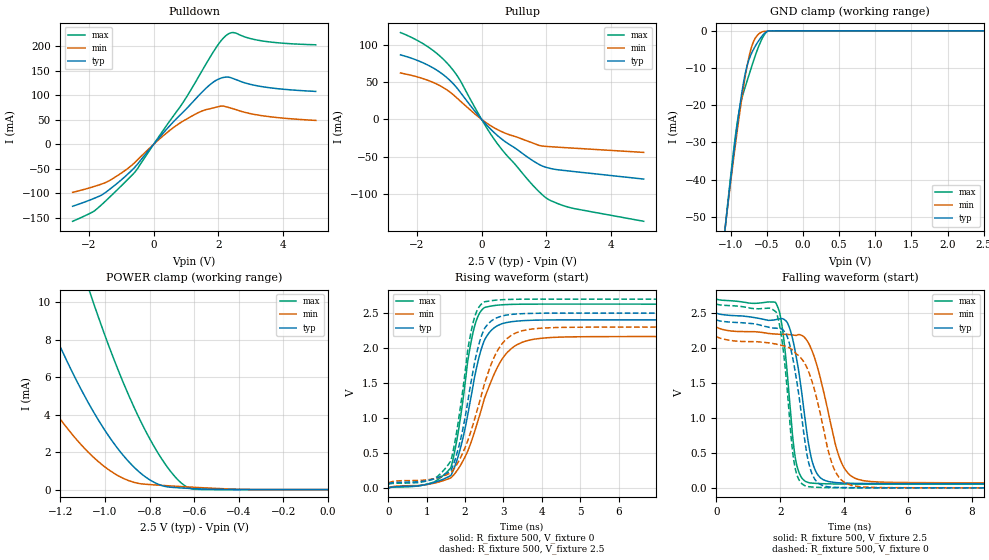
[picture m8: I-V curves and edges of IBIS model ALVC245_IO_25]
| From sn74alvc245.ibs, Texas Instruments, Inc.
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[Model]   ALVC245_IO_25
Model_type  I/O
Vinl=0.7
Vinh=1.7
Enable   Active-Low
Vref =   0
Rref =   500
Cref =   30p
Vmeas =   1.25
| variable   typ   min   max
C_comp   8.48pF   8.07pF   9.19pF
| C_pullup   10.89pF   8.22pF   13.18pF
| C_pulldown   14.36pF   8.64pF   20.00pF
| C_tri-state   8.48pF   8.07pF   9.19pF
[Temperature Range]   40   100   -40
| Ambient temperature   25   85   -40
[Voltage range]   2.5   2.3   2.7
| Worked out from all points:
|   slope of the pulldown table from 0 to 0.375 V, typ, clamps not added: 12.9 ohm
|   slope of the pullup table from 0 to 0.375 V, typ, clamps not added: 21.8 ohm
|   GND clamp passes 1 mA (typ) near -0.55 V on its own axis
|   POWER clamp passes 1 mA (typ) near -0.85 V on its own axis
|   rising waveform, R_fixture 500, V_fixture 0: 20-80 % time 555ps typ, 860ps min, 431ps max; typ from 0 V to 2.4 V
|   falling waveform, R_fixture 500, V_fixture 2.5: 20-80 % time 474ps typ, 713ps min, 327ps max; typ from 2.5 V to 0.061 V
|   rising waveform, R_fixture 500, V_fixture 2.5: 20-80 % time 524ps typ, 791ps min, 424ps max; typ from 0.061 V to 2.5 V
|   falling waveform, R_fixture 500, V_fixture 0: 20-80 % time 474ps typ, 740ps min, 328ps max; typ from 2.4 V to 0 V
[GND Clamp]
| ALVC245_IO_25
|   Voltage   I(typ)   I(min)   I(max)
-2.5V     -328.8mA   -310.3mA   -350mA
-1.085V   -54.4mA    -54.18mA   -54.48mA
-1.065V   -50.9mA    -50.92mA   -50.72mA
-970mV    -34.83mA   -35.87mA   -33.75mA
-910mV    -25.42mA   -26.89mA   -24.65mA
-865mV    -19.02mA   -20.55mA   -19.71mA
-805mV    -12.02mA   -12.92mA   -15.41mA
-750mV    -7.873mA   -7.224mA   -12.02mA
-705mV    -5.752mA   -3.933mA   -9.277mA
-585mV    -1.868mA   -456.6uA   -2.878mA
-470mV    -19.11uA   -68.6uA    -13.82uA
2.5V      86.77pA    69.93nA    14.99pA
[POWER Clamp]
| ALVC245_IO_25
|   Voltage   I(typ)   I(min)   I(max)
-2.5V     59.23mA    39.99mA    88.15mA
-1.535V   17.94mA    10.54mA    31.02mA
-1.515V   17.25mA    10.07mA    30.01mA
-1.295V   10.22mA    5.398mA    19.63mA
-1.165V   6.718mA    3.208mA    14.19mA
-1.06V    4.323mA    1.821mA    10.26mA
-950mV    2.303mA    801.1uA    6.651mA
-845mV    925.8uA    321uA      3.771mA
-745mV    216.5uA    225uA      1.628mA
-655mV    85.43uA    160.6uA    324.5uA
-595mV    47.22uA    120.6uA    14.24uA
-31.15fV  86.77pA    486.5pA    16.69pA
[Pulldown]
| ALVC245_IO_25
|   Voltage   I(typ)   I(min)   I(max)
-2.5V     -126.6mA   -98.21mA   -157.3mA
-1.855V   -110.9mA   -86.57mA   -137.2mA
-1.6V     -103.5mA   -81.07mA   -123.1mA
-1.075V   -77.02mA   -62.23mA   -89.88mA
-565mV    -45.65mA   -36.19mA   -55.64mA
265mV     20.74mA    15.8mA     25.76mA
895mV     64.89mA    46.9mA     84.31mA
1.77V     123.5mA    73.17mA    181.2mA
2.265V    137.4mA    76.13mA    223.8mA
2.48V     133.6mA    71.99mA    228mA
3.34V     117.8mA    58.51mA    211.3mA
5V        108mA      48.83mA    203.3mA
[Pullup]
| ALVC245_IO_25
|   Voltage   I(typ)   I(min)   I(max)
-2.5V     86.18mA    61.9mA     116mA
-1.655V   72.43mA    52.09mA    96.93mA
-1.31V    63.66mA    45.49mA    85.48mA
-1.005V   53.19mA    37.35mA    72.33mA
-680mV    37.48mA    25.32mA    53.38mA
35mV      -1.776mA   -1.163mA   -2.615mA
465mV     -20.76mA   -13.18mA   -31.26mA
1.51V     -53.32mA   -30.55mA   -84.78mA
1.965V    -63.86mA   -36.16mA   -104.3mA
2.33V     -67.33mA   -37.21mA   -112.4mA
2.77V     -69.48mA   -38.39mA   -118.5mA
5V        -79.91mA   -44.25mA   -136.4mA
[Ramp]
| ALVC245_IO_25
| variable   typ   min   max
dV/dt_r   1.44/5.79E-10   1.30/8.92E-10   1.58/4.51E-10
dV/dt_f   1.46/4.86E-10   1.34/7.27E-10   1.59/3.30E-10
R_load = 500
[Rising Waveform]
| ALVC245_IO_25
R_fixture =   500
C_fixture =   0
L_fixture =   0
V_fixture =   0
V_fixture_min = 0
V_fixture_max = 0
|   Time   V(typ)   V(min)   V(max)
0s        315pV      3.326nV    52.89pV
1.63ns    177.1mV    143.5mV    289.2mV
1.92ns    658.1mV    361.8mV    1.161V
2.065ns   1.035V     521.3mV    1.801V
2.255ns   1.606V     817.8mV    2.328V
2.5ns     2.107V     1.273V     2.577V
2.85ns    2.322V     1.734V     2.614V
3.485ns   2.392V     2.082V     2.628V
4.745ns   2.404V     2.16V      2.629V
50ns      2.403V     2.165V     2.629V
[Falling Waveform]
| ALVC245_IO_25
R_fixture =   500
C_fixture =   0
L_fixture =   0
V_fixture =   2.5
V_fixture_min = 2.3
V_fixture_max = 2.7
|   Time   V(typ)   V(min)   V(max)
0s        2.5V       2.3V       2.7V
1.88ns    2.409V     2.2V       2.631V
2.1ns     2.415V     2.196V     2.172V
2.295ns   2.284V     2.193V     1.244V
2.49ns    1.903V     2.18V      385.1mV
2.945ns   488.1mV    2.016V     70.21mV
3.25ns    147.4mV    1.583V     61.2mV
3.925ns   70.04mV    352.9mV    54.59mV
4.835ns   61.83mV    90.14mV    53.67mV
50ns      61.06mV    72.43mV    53.77mV
[Rising Waveform]
| ALVC245_IO_25
R_fixture =   500
C_fixture =   0
L_fixture =   0
V_fixture =   2.5
V_fixture_min = 2.3
V_fixture_max = 2.7
|   Time   V(typ)   V(min)   V(max)
0s        61.06mV    72.43mV    53.77mV
1.19ns    127.3mV    130.3mV    129.1mV
1.63ns    246.3mV    215.8mV    387.4mV
1.915ns   774.3mV    471.4mV    1.3V
2.225ns   1.728V     941.2mV    2.399V
2.48ns    2.249V     1.44V      2.654V
2.785ns   2.423V     1.902V     2.685V
3.325ns   2.487V     2.217V     2.698V
4.635ns   2.5V       2.297V     2.7V
50ns      2.5V       2.3V       2.7V
[Falling Waveform]
| ALVC245_IO_25
R_fixture =   500
C_fixture =   0
L_fixture =   0
V_fixture =   0
V_fixture_min = 0
V_fixture_max = 0
|   Time   V(typ)   V(min)   V(max)
0s        2.403V     2.165V     2.629V
1.875ns   2.284V     2.056V     2.514V
2.09ns    2.257V     2.033V     1.993V
2.355ns   1.938V     1.982V     661.9mV
2.46ns    1.687V     1.938V     302.3mV
2.905ns   332.8mV    1.643V     16.14mV
3.18ns    72.84mV    1.209V     7.544mV
3.695ns   8.235mV    263.3mV    1.392mV
4.52ns    1.123mV    14.96mV    -40.02uV
50ns      799.6nV    -1.135uV   382.4nV
